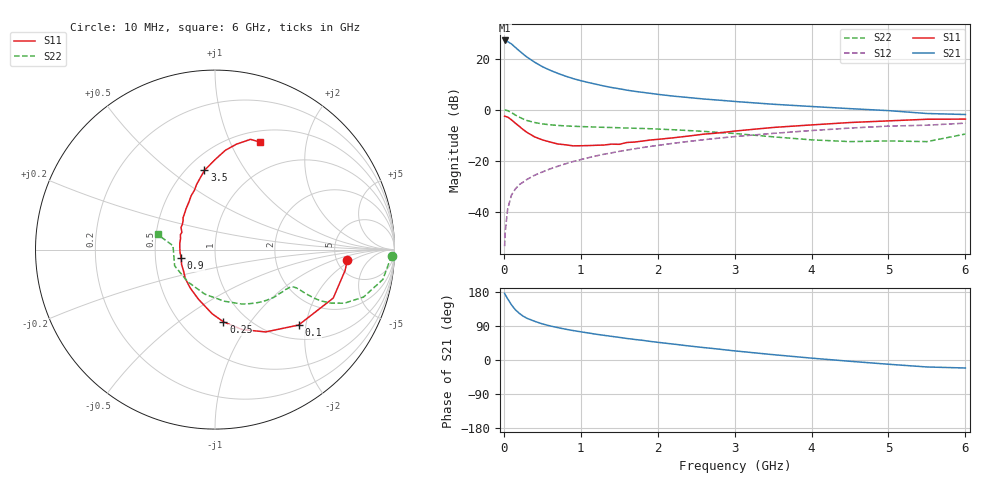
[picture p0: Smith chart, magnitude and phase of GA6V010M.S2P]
! Infineon Technologies  Discrete & RF Semiconductors
! BF775
! Si NPN RF Bipolar Junction Transistor in SOT23
! VCE = 6 V  IC = 10 mA
! Common Emitter S-Parameters:  May  1996
# GHz  S  MA  R  50
!  f  S11  S21  S12  S22
! GHz  MAG  ANG  MAG  ANG  MAG  ANG  MAG  ANG
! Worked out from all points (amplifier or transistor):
!   36 points, 10 MHz to 6 GHz, reference 50 ohm
!   highest |S21| = 27.1 dB at 10 MHz (marker M1)
!   |S21| within 3 dB of that: start of sweep to 160.1 MHz
!   unconditionally stable (mu >= 1): 613.7 MHz to 2.947 GHz
!   at 250 MHz: K = 0.67, MSG = 25.1 dB, |S12| = -28.5 dB
!   at 1.4 GHz: K = 1.10, MAG = 10.9 dB, |S12| = -17.0 dB
!   at 6 GHz: K = 0.91, MSG = 1.7 dB, |S12| = -5.3 dB
!   S11 on the Smith chart (normalised r, x): 10 MHz: 6.21, -1.66; 100 MHz: 1.31, -1.82; 250 MHz: 0.78, -0.75; 900 MHz: 0.68, -0.07; 3.5 GHz: 0.61, +0.67; 6 GHz: 0.63, +1.30
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0.01  0.7392 -4.7  22.58 175.8  0.0021 90.4  0.9864 -2.0
0.02  0.7342 -9.1  22.27 171.8  0.0043 85.8  0.9734 -4.1
0.05  0.712 -22.3  21.48 161.3  0.0113 79.8  0.9498 -10.1
0.1  0.6272 -42.1  19.26 145.5  0.0212 71.7  0.8689 -17.7
0.15  0.5385 -58.4  16.48 132.5  0.0278 66.1  0.7803 -22.5
0.2  0.4701 -71.3  14.19 123.4  0.0337 64.4  0.7103 -24.8
0.25  0.4054 -83.3  12.24 115.8  0.0377 62.5  0.6528 -25.9
0.3  0.3576 -92.6  10.7 110.1  0.0426 63.1  0.61 -26.1
0.4  0.291 -108.6  8.466 102.2  0.0516 63.3  0.5567 -25.8
0.5  0.2548 -122.7  6.929 95.3  0.0597 64.3  0.523 -25.4
0.6  0.2311 -135.7  5.897 90.0  0.0685 65.0  0.5026 -25.2
0.7  0.2115 -146.1  5.129 85.5  0.0771 65.3  0.4882 -25.4
0.9  0.1942 -165.5  4.044 77.7  0.0956 65.4  0.4701 -26.4
1.1  0.1966 176.0  3.382 71.3  0.1139 65.2  0.4583 -28.3
1.3  0.2014 162.4  2.894 65.2  0.1328 64.1  0.4479 -30.4
1.6  0.2261 146.9  2.4 56.8  0.1605 62.3  0.4338 -34.5
2.2  0.2789 125.3  1.833 42.1  0.2176 57.3  0.4019 -44.8
3  0.3783 105.6  1.44 24.1  0.2949 48.9  0.3392 -63.5
3.5  0.4453 97.6  1.27 14.1  0.341 43.0  0.2918 -80.0
4.5  0.5568 84.0  1.041 -3.4  0.4332 30.3  0.2352 -130.0
5.5  0.6451 72.2  0.836 -18.4  0.493 15.4  0.235 174.7
6  0.6493 67.3  0.799 -21.1  0.541 11.3  0.3311 165.2
